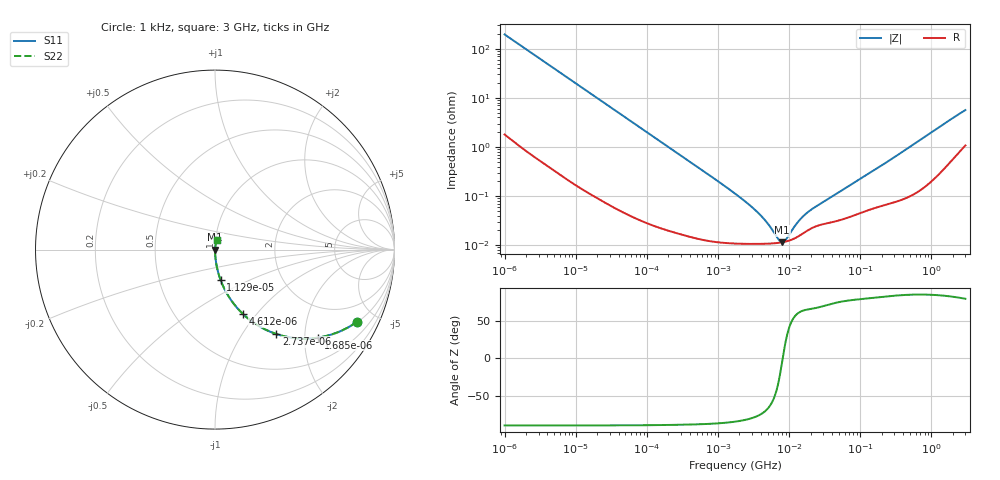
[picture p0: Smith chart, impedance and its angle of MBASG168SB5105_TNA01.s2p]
! MBASG168SB5105_TNA01  S-PARAMETER MODEL  ( Standard Model )
! Model Generated by TAIYO YUDEN Corporation (http://www.ty-top.com)
! Version 2.0
! TAIYO YUDEN Control No. 230906
! Copyright(c) 2012 TAIYO YUDEN CO.,LTD. All Rights Reserved.
! Product Description (link to TY-COMPAS)
! https://ds.yuden.co.jp/TYCOMPAS/or/detail?pn=MBASG168SB5105KTNA01&u=M
! Products Name : Multilayer Ceramic Capacitors
! Characteristics :
!  Capacitance : 1 [uF] , Rated Voltage : 35 [V] , TCC : X5R
!  Case Size : 1.6 x 0.8 / 0.063 x 0.031 [mm/inch] , Thickness : 0.8 / 0.031 [mm/inch]
!  (Conditions: Temperature = 25 [degC] , DC Bias Voltage = 0 [V])
! External Node Assignments :
!  1  o---| |---o  2
! GND o---------o GND
! Frequency Range : 1kHz  -  3GHz  [ 401 STEP ]
# MHZ S RI R 50
! Freq[MHz].  S11 Real  S11 Imag  S21 Real  S21 Imag  S12 Real  S12 Imag  S22 Real  S22 Imag
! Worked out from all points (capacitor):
!   401 points, 1 kHz to 3 GHz, reference 50 ohm
!   read as one part in series: C = 813 nF near 1.077 kHz
!   lowest |Z| = 11.5 mohm at 7.989 MHz (marker M1)
!   series resonance near 8.123 MHz, so ESL is about 470 pH
!   S11 on the Smith chart (normalised r, x): 1 kHz: 1.04, -3.91; 1.685 kHz: 1.02, -2.32; 2.737 kHz: 1.01, -1.44; 4.612 kHz: 1.01, -0.85; 11.29 kHz: 1.00, -0.35; 3 GHz: 1.02, +0.11
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0.001  0.7902 -0.4026  0.2098 0.4026  0.2098 0.4026  0.7902 -0.4026
0.001685  0.5741 -0.4902  0.4259 0.4902  0.4259 0.4902  0.5741 -0.4902
0.002737  0.3412 -0.47  0.6588 0.47  0.6588 0.47  0.3412 -0.47
0.004612  0.1562 -0.3589  0.8438 0.3589  0.8438 0.3589  0.1562 -0.3589
0.006951  0.0764 -0.2615  0.9236 0.2615  0.9236 0.2615  0.0764 -0.2615
0.011286  0.0311 -0.1695  0.9689 0.1695  0.9689 0.1695  0.0311 -0.1695
0.01216  0.0271 -0.1581  0.9729 0.1581  0.9729 0.1581  0.0271 -0.1581
0.033275  0.00415 -0.0595  0.9959 0.0595  0.9959 0.0595  0.00415 -0.0595
0.147855  0.000411 -0.0135  0.9996 0.0135  0.9996 0.0135  0.000411 -0.0135
1.732051  0.000109 -0.00112  0.9999 0.00112  0.9999 0.00112  0.000109 -0.00112
2.709407  0.000107 -0.000668  0.9999 0.000668  0.9999 0.000668  0.000107 -0.000668
3.789741  0.000106 -0.000421  0.9999 0.000421  0.9999 0.000421  0.000106 -0.000421
5.106836  0.000108 -0.000242  0.9999 0.000242  0.9999 0.000242  0.000108 -0.000242
7.143107  0.000112 -6.52e-05  0.9999 6.52e-05  0.9999 6.52e-05  0.000112 -6.52e-05
7.988506  0.000115 -8.41e-06  0.9999 8.41e-06  0.9999 8.41e-06  0.000115 -8.41e-06
8.933959  0.000118 4.85e-05  0.9999 -4.85e-05  0.9999 -4.85e-05  0.000118 4.85e-05
12.03889  0.000139 0.000204  0.9999 -0.000204  0.9999 -0.000204  0.000139 0.000204
14.50609  0.000162 0.000304  0.9998 -0.000304  0.9998 -0.000304  0.000162 0.000304
21.06097  0.000225 0.000498  0.9998 -0.000498  0.9998 -0.000498  0.000225 0.000498
256.0921  0.000724 0.00526  0.9993 -0.00526  0.9993 -0.00526  0.000724 0.00526
1714.862  0.00546 0.033  0.9945 -0.033  0.9945 -0.033  0.00546 0.033
3000  0.0136 0.0541  0.9864 -0.0541  0.9864 -0.0541  0.0136 0.0541
